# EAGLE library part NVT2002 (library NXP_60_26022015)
Bidirectional voltage level translator for open-drain and push-pull applications The NVT2001/02 are bidirectional voltage level translators operational from 1.0 V to 3.6 V (Vref(A)) and 1.8 V to 5.5 V (Vref(B)), which allow bidirectional voltage translations between 1.0 V and 5 V without the need for a direction pin in open-drain or push-pull applications. Bit widths ranging from 1-bit or 2-bit are offered for level translation application with transmission speeds 33 MHz for an open-drain system with a 50 pF capacitance and a pull-up of 197. When the An or Bn port is LOW, the clamp is in the ON-state and a low resistance connection exists between the An and Bn ports. The low ON-state resistance (Ron) of the switch allows connections to be made with minimal propagation delay. Assuming the higher voltage is on the Bn port when the Bn port is HIGH, the voltage on the An port is limited to the voltage set by VREFA. When the An port is HIGH, the Bn port is pulled to the drain pull-up supply voltage (Vpu(D)) by the pull-up resistors. This functionality allows a seamless translation between higher and lower voltages selected by the user without the need for directional control. When EN is HIGH, the translator switch is on, and the An I/O are connected to the Bn I/O, respectively, allowing bidirectional data flow between ports. When EN is LOW, the translator switch is off, and a high-impedance state exists between ports. The EN input circuit is designed to be supplied by Vref(B). To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
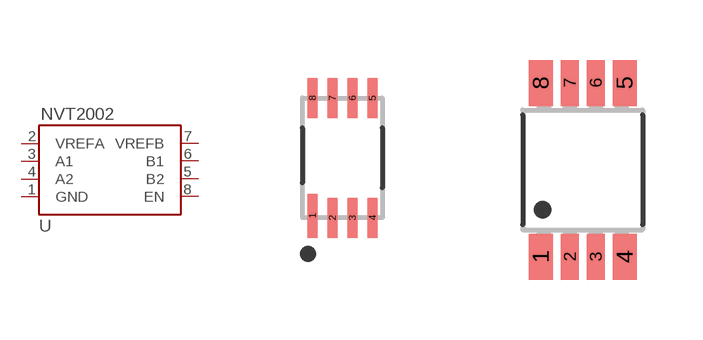
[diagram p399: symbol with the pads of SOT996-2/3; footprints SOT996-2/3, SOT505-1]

Designator prefix U

## NVT2002GD  [SOT996-2/3]
1  GND  pwr
2  VREFA  pwr
3  A1
4  A2
5  B2
6  B1
7  VREFB  pwr
8  EN  in

## NVT2002DP  [SOT505-1]
Pads as for SOT996-2/3

## Footprint SOT996-2/3 (pad centres in mm)
SOT996-2/3 XSON8U: plastic extremely thin small outline package; no leads;8 terminals; UTLP based; body 3 x 2 x 0.5 mm JEDEC: IEC: -- JEITA: --
smd 0.25 x 1.1: 1 -0.75,-1.45
smd 0.25 x 1: 2 -0.25,-1.5; 3 0.25,-1.5; 4 0.75,-1.5; 5 0.75,1.5; 6 0.25,1.5; 7 -0.25,1.5; 8 -0.75,1.5

## Footprint SOT505-1 (pad centres in mm)
SOT505-1 TSSOP8: plastic thin shrink small outline package; 8 leads; body width 3 mm JEDEC: -- IEC: --
smd 0.6 x 1.15: 1 -1.05,-2.175; 4 1.05,-2.175; 5 1.05,2.175; 8 -1.05,2.175
smd 0.45 x 1.15: 2 -0.325,-2.175; 3 0.325,-2.175; 6 0.325,2.175; 7 -0.325,2.175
